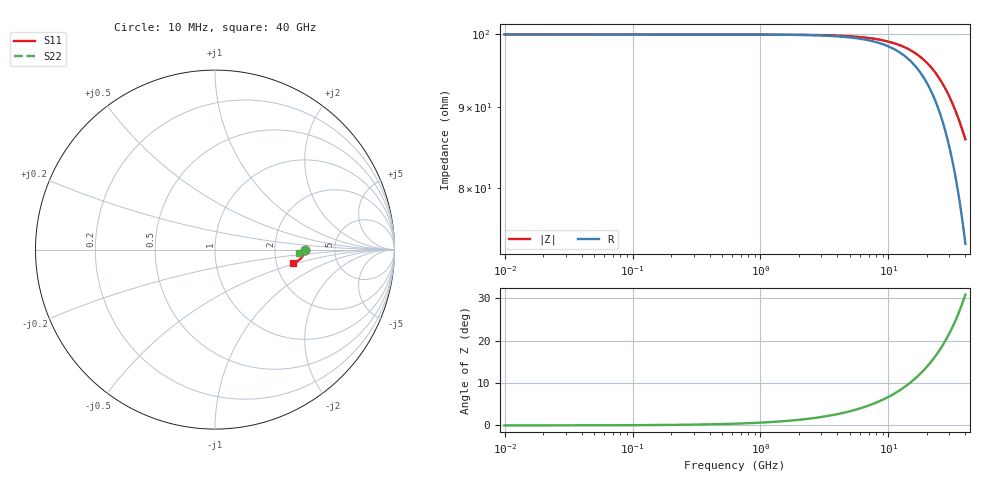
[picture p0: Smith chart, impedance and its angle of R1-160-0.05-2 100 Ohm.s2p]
!version-1
!date-04.2022
# MHz S RI R 50
!Freq ReS11 ImS11 ReS21 ImS21 ReS12 ImS12 ReS22 ImS22
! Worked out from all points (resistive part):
!   801 points, 10 MHz to 40 GHz, reference 50 ohm
!   read as one part in series: R = 100 ohm at 210 MHz
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10  0.5 -2.24e-05  0.5 -5.52e-05  0.5 -5.52e-05  0.5 -6.45e-06
210  0.5 -0.000469  0.5 -0.00116  0.5 -0.00116  0.5 -0.000135
3360  0.4995 -0.0075  0.5001 -0.0186  0.5001 -0.0186  0.4998 -0.00217
6710  0.4982 -0.0149  0.5002 -0.0372  0.5002 -0.0372  0.4991 -0.00431
10060  0.4959 -0.0223  0.5005 -0.056  0.5005 -0.056  0.498 -0.00642
13360  0.4927 -0.0294  0.5008 -0.075  0.5008 -0.075  0.4965 -0.00845
15060  0.4908 -0.033  0.501 -0.0849  0.501 -0.0849  0.4956 -0.00947
16710  0.4886 -0.0365  0.5012 -0.0947  0.5012 -0.0947  0.4946 -0.0104
20010  0.4836 -0.0432  0.5016 -0.1147  0.5016 -0.1147  0.4922 -0.0123
21660  0.4808 -0.0464  0.5018 -0.125  0.5018 -0.125  0.4909 -0.0132
23360  0.4777 -0.0497  0.502 -0.1358  0.502 -0.1358  0.4894 -0.0141
25060  0.4743 -0.0528  0.5021 -0.1468  0.5021 -0.1468  0.4878 -0.0149
26710  0.4707 -0.0558  0.5021 -0.1578  0.5021 -0.1578  0.4861 -0.0157
28410  0.4669 -0.0587  0.5022 -0.1694  0.5022 -0.1694  0.4843 -0.0165
30110  0.4628 -0.0615  0.5021 -0.1812  0.5021 -0.1812  0.4824 -0.0172
31760  0.4586 -0.0641  0.5019 -0.1931  0.5019 -0.1931  0.4805 -0.0178
33360  0.4543 -0.0664  0.5017 -0.2049  0.5017 -0.2049  0.4785 -0.0184
34810  0.4503 -0.0684  0.5013 -0.2158  0.5013 -0.2158  0.4767 -0.0189
36260  0.4461 -0.0703  0.5008 -0.2271  0.5008 -0.2271  0.4748 -0.0193
38010  0.4409 -0.0724  0.5 -0.2411  0.5 -0.2411  0.4724 -0.0198
39810  0.4353 -0.0744  0.499 -0.2559  0.499 -0.2559  0.4699 -0.0202
40000  0.4347 -0.0746  0.4988 -0.2575  0.4988 -0.2575  0.4697 -0.0203
